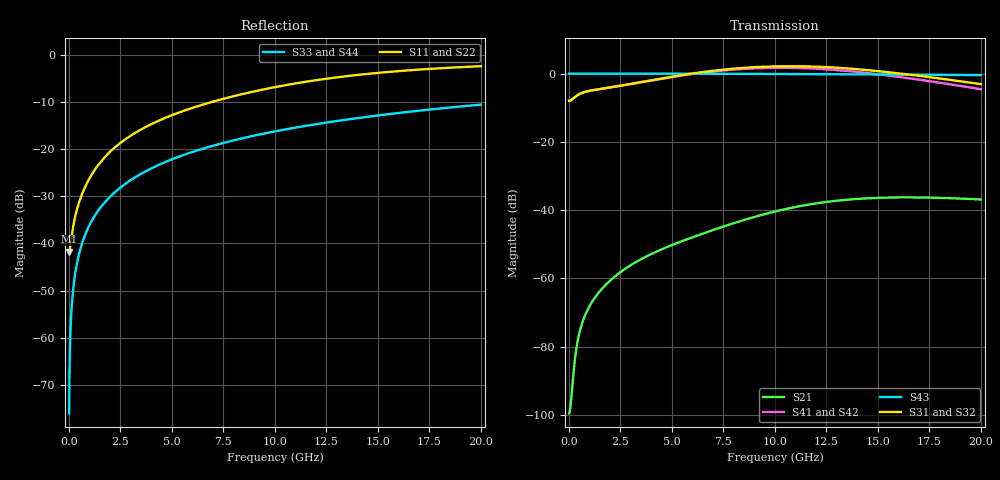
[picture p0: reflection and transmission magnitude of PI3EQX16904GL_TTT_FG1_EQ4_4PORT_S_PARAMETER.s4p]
! NPort=4 DATA=2000 NOISE=0 GROUPDELAY=0 COMPLEX_DATAFORMAT=POLAR
! NumOfBlock=1 NumOfParam=0
! .MODEL Smodel S TSTONEFILE=PI3EQX16904GL_TTT_FG1_EQ4_4PORT_S_PARAMETER.s4p TYPE=S
!  -- The above .MODEL line can be used for the S element in the netlist.
! The s parameter is extracted from the linear redriver, it is not bi-directional; only s(4,1)s(4,2) and s(3,1)s(3,2)
! should be the insertion loss
!Port definition:
!Port1 = input+
!Port2 = input-
!Port3 = output+
!Port4 = output-
# Hz S MA R  50
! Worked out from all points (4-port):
!   2000 points, 10 MHz to 20 GHz, reference 50 ohm
!   strongest paths, dB at 10 MHz, 5.01 GHz, 10.01 GHz, 15.01 GHz, 20 GHz:
!     S31: -8.0, -0.9, 2.1, 0.7, -3.1
!     S43: 0.0, 0.0, -0.1, -0.3, -0.4
!     S32: -8.0, -1.1, 1.8, 0.4, -3.4
!     S41: -8.0, -1.0, 1.7, -0.2, -4.6
!     S42: -8.0, -1.2, 1.4, -0.5, -4.9
!     S21: -99.6, -50.2, -40.4, -36.4, -36.9
!   lowest |S11| = -41.7 dB at 10 MHz (marker M1), VSWR 1.02, Z = 49.2 - j0.0603 ohm
!   |S11| at or under -10 dB: start of sweep to 6.893 GHz
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1e7  0.008182 -175.7  1.05e-05 7.7  0 0.0  0 0.0
     1.05e-05 7.7  0.008182 -175.7  0 0.0  0 0.0
     0.3996 0.4  0.3996 -179.6  0.0001571 -90.0  1 -0.0
     0.3996 -179.6  0.3996 0.4  1 -0.0  0.0001571 -90.0
6.2e8  0.03268 -112.4  0.0002097 114.5  0 0.0  0 0.0
       0.0002097 114.5  0.03268 -112.4  0 0.0  0 0.0
       0.5193 8.3  0.5187 -171.9  0.009738 -90.6  0.9999 -0.6
       0.5192 -172.8  0.5186 7.0  0.9999 -0.6  0.009738 -90.6
2.97e9  0.1383 -101.5  0.001537 101.0  0 0.0  0 0.0
        0.001536 100.9  0.1383 -101.6  0 0.0  0 0.0
        0.7029 -7.2  0.6965 171.7  0.0466 -92.8  0.9988 -2.7
        0.6998 167.4  0.6934 -13.6  0.9988 -2.7  0.0466 -92.8
6.69e9  0.307 -106.2  0.004775 84.8  0 0.0  0 0.0
        0.004738 85.0  0.307 -106.2  0 0.0  0 0.0
        1.071 -48.1  1.04 131.0  0.1045 -96.2  0.9941 -6.0
        1.048 120.1  1.016 -60.9  0.9941 -6.0  0.1045 -96.2
1.009e10  0.4612 -113.1  0.009756 59.5  0 0.0  0 0.0
          0.00966 60.2  0.4607 -113.1  0 0.0  0 0.0
          1.278 -99.8  1.237 79.7  0.1564 -99.4  0.9867 -9.0
          1.216 62.7  1.177 -117.8  0.9867 -9.0  0.1564 -99.4
1.422e10  0.6236 -123.4  0.01481 15.9  0 0.0  0 0.0
          0.01471 17.1  0.6228 -123.4  0 0.0  0 0.0
          1.144 -164.7  1.107 14.9  0.2176 -103.1  0.9741 -12.6
          1.041 -8.7  1.008 171.0  0.9741 -12.6  0.2176 -103.1
2e10  0.7641 -136.0  0.01431 -34.2  0 0.0  0 0.0
      0.01429 -32.5  0.7638 -136.0  0 0.0  0 0.0
      0.7005 117.8  0.6778 -62.4  0.2986 -108.1  0.9506 -17.4
      0.5898 -94.1  0.5707 85.7  0.9506 -17.4  0.2986 -108.1
